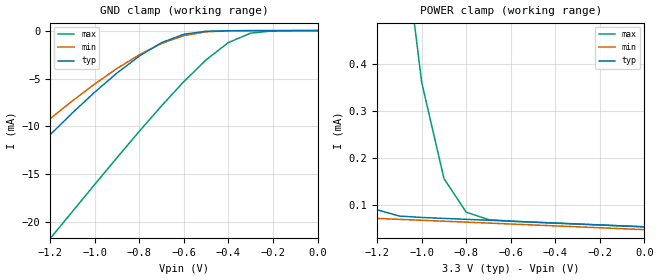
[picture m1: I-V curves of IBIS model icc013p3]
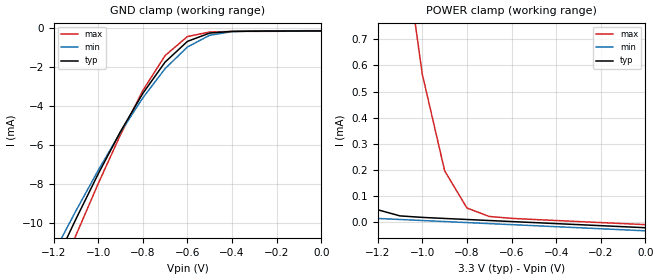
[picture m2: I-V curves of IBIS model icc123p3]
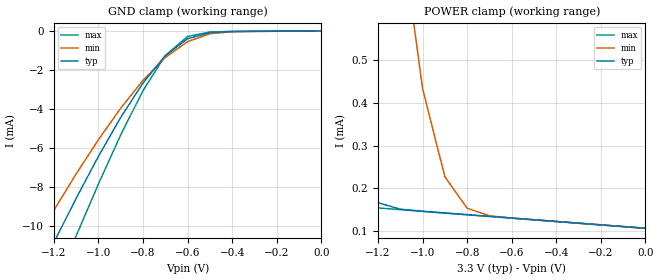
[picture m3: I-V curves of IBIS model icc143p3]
[IBIS ver]   2.1
[File name]   mpc9893.ibs
[File Rev]   2.2 {April 29, 2002}
[Date]   December 13th, 2002
[Disclaimer]   This information is for modeling purposes only
|   and is not guaranteed.
[Source]   Timing Solutions Operations
[Copyright]   Copyright 2001, Motorola Incorporated,
|   all rights reserved.
| Component MPC9893 for 3.3V Application!
[Component]   MPC9893_3p3
[Manufacturer]   Motorola
[Package]
|   typ   min   max
R_pkg   0.048   .038   0.053
L_pkg   6.045nH   5.084nH   7.950nH
C_pkg   0.813pF   0.560pF   1.157pF
[Pin]   signal_name model_name R_pin L_pin   C_pin
2   QFB   occ013p3   0.04   0.35nH   0.053pF
3   FB   icc013p3   0.04   0.35nH   0.053pF
4   MANB/A   icc123p3   0.04   0.35nH   0.053pF
6   CLK0   icc013p3   0.04   0.35nH   0.053pF
7   CLK1   icc013p3   0.04   0.35nH   0.053pF
9   ALARMB/0   occ013p3   0.04   0.35nH   0.053pF
10   ALARMB/1   occ013p3   0.04   0.35nH   0.053pF
11   CLK_IND   occ013p3   0.04   0.35nH   0.053pF
14   QB5   occ013p3   0.04   0.35nH   0.053pF
15   QB4   occ013p3   0.04   0.35nH   0.053pF
18   QB3   occ013p3   0.04   0.35nH   0.053pF
19   QB2   occ013p3   0.04   0.35nH   0.053pF
22   QB1   occ013p3   0.04   0.35nH   0.053pF
23   QB0   occ013p3   0.04   0.35nH   0.053pF
26   OEB/MR   icc143p3   0.04   0.35nH   0.053pF
27   FSEL3   icc143p3   0.04   0.35nH   0.053pF
28   FSEL2   icc143p3   0.04   0.35nH   0.053pF
30   FSEL1   icc143p3   0.04   0.35nH   0.053pF
31   FSEL0   icc143p3   0.04   0.35nH   0.053pF
33   PLL_ENB   icc143p3   0.04   0.35nH   0.053pF
34   REF_SEL   icc143p3   0.04   0.35nH   0.053pF
35   ALARMB_RST  icc123p3   0.04   0.35nH   0.053pF
38   QA0   occ013p3   0.04   0.35nH   0.053pF
39   QA1   occ013p3   0.04   0.35nH   0.053pF
42   QA2   occ013p3   0.04   0.35nH   0.053pF
43   QA3   occ013p3   0.04   0.35nH   0.053pF
46   QA4   occ013p3   0.04   0.35nH   0.053pF
47   QA5   occ013p3   0.04   0.35nH   0.053pF
|Component MPC9893 for 2.5V Application!
[Component]   MPC9893_2p5
[Manufacturer]   Motorola
[Package]
|   typ   min   max
R_pkg   0.048   .038   0.053
L_pkg   6.045nH   5.084nH   7.950nH
C_pkg   0.813pF   0.560pF   1.157pF
[Pin]   signal_name model_name R_pin L_pin   C_pin
2   QFB   occ012p5   0.04   0.35nH   0.053pF
3   FB   icc012p5   0.04   0.35nH   0.053pF
4   MANB/A   icc122p5   0.04   0.35nH   0.053pF
6   CLK0   icc012p5   0.04   0.35nH   0.053pF
7   CLK1   icc012p5   0.04   0.35nH   0.053pF
9   ALARMB/0   occ012p5   0.04   0.35nH   0.053pF
10   ALARMB/1   occ012p5   0.04   0.35nH   0.053pF
11   CLK_IND   occ012p5   0.04   0.35nH   0.053pF
14   QB5   occ012p5   0.04   0.35nH   0.053pF
15   QB4   occ012p5   0.04   0.35nH   0.053pF
18   QB3   occ012p5   0.04   0.35nH   0.053pF
19   QB2   occ012p5   0.04   0.35nH   0.053pF
22   QB1   occ012p5   0.04   0.35nH   0.053pF
23   QB0   occ012p5   0.04   0.35nH   0.053pF
26   OEB/MR   icc142p5   0.04   0.35nH   0.053pF
27   FSEL3   icc142p5   0.04   0.35nH   0.053pF
28   FSEL2   icc142p5   0.04   0.35nH   0.053pF
30   FSEL1   icc142p5   0.04   0.35nH   0.053pF
31   FSEL0   icc142p5   0.04   0.35nH   0.053pF
33   PLL_ENB   icc142p5   0.04   0.35nH   0.053pF
34   REF_SEL   icc142p5   0.04   0.35nH   0.053pF
35   ALARMB_RST  icc122p5   0.04   0.35nH   0.053pF
38   QA0   occ012p5   0.04   0.35nH   0.053pF
39   QA1   occ012p5   0.04   0.35nH   0.053pF
42   QA2   occ012p5   0.04   0.35nH   0.053pF
43   QA3   occ012p5   0.04   0.35nH   0.053pF
46   QA4   occ012p5   0.04   0.35nH   0.053pF
47   QA5   occ012p5   0.04   0.35nH   0.053pF
| Models and submodels in the file (8): icc013p3 (Input), icc123p3 (Input), icc143p3 (Input), occ013p3 (Output), icc012p5 (Input), icc122p5 (Input), icc142p5 (Input), occ012p5 (Output)
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|This is a Model of an Input with a 25,000 ohm Pull_down at 3.3V
[Model]   icc013p3
Model_type   Input
Polarity   Non-Inverting
Vmeas=1.5
Vinl=0.8
Vinh=2.0
| Variable   typ   min   max
C_comp   5p   5p   5p
[Temperature Range]   27.00   100.00   -45.00
[Power Clamp Reference]   3.30V   3.0V   3.6V
[Gnd Clamp Reference]   0.000V   0.000V   0.000V
[Voltage Range]   3.30V   3.0V   3.6V
[Pulldown Reference]   0.000V   0.000V   0.000V
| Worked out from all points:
|   GND clamp passes 1 mA (typ) near -0.67 V on its own axis
|   POWER clamp passes 1 mA (typ) near -1.50 V on its own axis
[GND_clamp]
|   voltage   I(typ)   I(mim)   I(max)
-3.3V     -64.02mA   -56.37mA   -80.44mA
-1.8V     -25.56mA   -21.69mA   -38.72mA
-1.7V     -23.03mA   -19.5mA    -35.89mA
-1.6V     -20.51mA   -17.33mA   -33.05mA
-1.2V     -10.84mA   -9.179mA   -21.67mA
-1.1V     -8.57mA    -7.315mA   -18.85mA
-900mV    -4.418mA   -3.945mA   -13.24mA
-700mV    -1.251mA   -1.342mA   -7.834mA
-600mV    -381.4uA   -529.5uA   -5.315mA
-400mV    -13.34uA   -24.07uA   -1.246mA
-300mV    -6.264uA   -7.567uA   -268.1uA
1.97fV    -11.82pA   -304.9pA   -5.993uA
[POWER_clamp]
|   voltage   I(typ)   I(mim)   I(max)
-3.3V     24.4mA     18.52mA    23.82mA
-2.1V     7.098mA    708uA      9.272mA
-2V       5.867mA    235uA      8.195mA
-1.9V     4.703mA    99.99uA    7.152mA
-1.4V     474.5uA    75.62uA    2.627mA
-1.3V     176.1uA    73.63uA    1.907mA
-1.2V     89.81uA    71.64uA    1.272mA
-1.1V     76.66uA    69.65uA    744.2uA
-1V       73.7uA     67.66uA    360.8uA
-900mV    71.64uA    65.67uA    156.3uA
-800mV    69.65uA    63.68uA    84.81uA
1.97fV    53.73uA    47.76uA    53.73uA
|This model is an Input with a 25,000 ohm Pull_up at 3.3V
[Model]   icc123p3
Model_type   Input
Polarity   Non-Inverting
Vmeas=1.5
Vinl=.8
Vinh=2.0
| Variable   typ   min   max
C_comp   5p   5p   5p
[Temperature Range]   27.00   100.00   -45.00
[Power Clamp Reference]   3.30V   3.00V   3.60V
[Gnd Clamp Reference]   0.000V   0.000V   0.000V
[Voltage Range]   3.30V   3.00V   3.60V
[Pulldown Reference]   0.000V   0.000V   0.000V
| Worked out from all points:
|   GND clamp passes 1 mA (typ) near -0.63 V on its own axis
|   POWER clamp passes 1 mA (typ) near -1.46 V on its own axis
[GND_clamp]
|   voltage   I(typ)   I(mim)   I(max)
-3.3V     -67.3mA    -63.37mA   -72.33mA
-1.2V     -12.25mA   -11.58mA   -13.41mA
-1.1V     -9.822mA   -9.397mA   -10.66mA
-1V       -7.495mA   -7.309mA   -7.997mA
-900mV    -5.313mA   -5.354mA   -5.475mA
-800mV    -3.351mA   -3.58mA    -3.204mA
-700mV    -1.737mA   -2.073mA   -1.402mA
-600mV    -671.6uA   -960.6uA   -422.5uA
-500mV    -242.1uA   -355.2uA   -187.1uA
-400mV    -155.8uA   -168.6uA   -159.6uA
1.97fV    -130.7uA   -118.8uA   -142.6uA
[POWER_clamp]
|   voltage   I(typ)   I(min)   I(max)
-3.3V     27.53mA    23.85mA    31.14mA
-1.9V     5.629mA    1.476mA    10.03mA
-1.8V     4.372mA    654.1uA    8.7mA
-1.7V     3.212mA    179.2uA    7.413mA
-1.5V     1.28mA     24.5uA     5.006mA
-1.4V     591.2uA    19.82uA    3.906mA
-1.3V     181.7uA    15.84uA    2.889mA
-1.1V     21.73uA    7.921uA    1.18mA
-1V       15.97uA    3.96uA     565.8uA
-900mV    11.89uA    3.897pA    195.3uA
-800mV    7.921uA    -3.96uA    51.97uA
1.97fV    -23.76uA   -35.64uA   -11.88uA
|This model is an Input with a 25,000 ohm Pull_down at 3.3V
[Model]   icc143p3
Model_type   Input
Polarity   Non-Inverting
Vmeas=1.5
Vinl=.8
Vinh=2.0
| Variable   typ   min   max
C_comp   5p   5p   5p
[Temperature Range]   27.00   100.00   -45.00
[Voltage Range]   3.30V   3.00V   3.60V
[Pulldown Reference]   0.000V   0.000V   0.000V
[Power Clamp Reference]   3.30V   3.0V   3.6V
[Gnd Clamp Reference]   0.000V   0.000V   0.000V
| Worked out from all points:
|   GND clamp passes 1 mA (typ) near -0.67 V on its own axis
|   POWER clamp passes 1 mA (typ) near -1.48 V on its own axis
[GND_clamp]
|   voltage   I(typ)   I(mim)   I(max)
-3.3V     -64.09mA   -56.43mA   -72.19mA
-1.3V     -13.21mA   -11.15mA   -16.06mA
-1.2V     -10.86mA   -9.203mA   -13.26mA
-1.1V     -8.591mA   -7.337mA   -10.52mA
-1V       -6.433mA   -5.579mA   -7.854mA
-900mV    -4.435mA   -3.962mA   -5.332mA
-800mV    -2.671mA   -2.531mA   -3.061mA
-700mV    -1.265mA   -1.356mA   -1.26mA
-600mV    -393.2uA   -541.3uA   -279.9uA
-500mV    -78.4uA    -139.9uA   -44.53uA
-400mV    -21.23uA   -31.95uA   -17.01uA
1.97fV    -11.82pA   -304.9pA   -3.647pA
[POWER_clamp]
|   voltage   I(typ)   I(min)   I(max)
-3.3V     24.52mA    23.94mA    23.99mA
-1.8V     3.707mA    6.236mA    796.6uA
-1.7V     2.716mA    5.273mA    321.7uA
-1.6V     1.838mA    4.359mA    184.7uA
-1.4V     555.3uA    2.707mA    162.4uA
-1.3V     254.9uA    1.986mA    158.4uA
-1.2V     166.6uA    1.349mA    154.5uA
-1.1V     151.5uA    819uA      150.5uA
-1V       146.6uA    433.7uA    146.5uA
-900mV    142.6uA    227.2uA    142.6uA
-800mV    138.6uA    153.8uA    138.6uA
1.97fV    106.9uA    106.9uA    106.9uA
